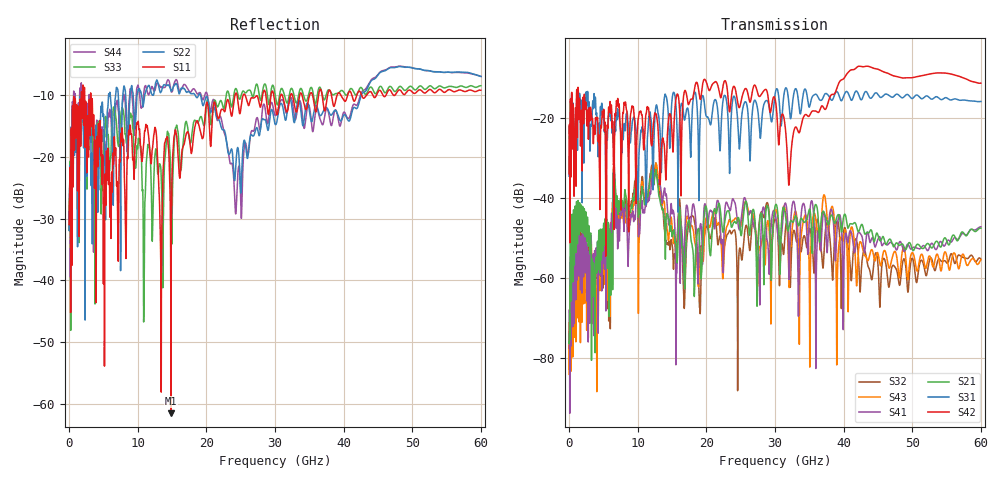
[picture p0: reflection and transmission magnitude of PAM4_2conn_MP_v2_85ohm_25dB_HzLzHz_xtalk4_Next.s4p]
! Info: Touchstone file created by Circ.  Input file=FAB50GbE_2conn_Midplane_Examax_Topo2_v2_85ohm_25dB_HzLzHz.circ
# Hz S RI R 50
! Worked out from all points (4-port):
!   6000 points, 10 MHz to 60 GHz, reference 50 ohm
!   strongest paths, dB at 10 MHz, 15.01 GHz, 30.01 GHz, 45.01 GHz, 60 GHz:
!     S42: -34.0, -24.0, -15.3, -7.9, -11.4
!     S31: -34.6, -15.5, -14.2, -14.2, -16.0
!     S21: -76.0, -49.8, -42.2, -49.4, -47.6
!     S41: -68.1, -44.1, -43.8, -50.4, -47.3
!     S43: -71.3, -47.6, -43.1, -53.9, -55.5
!     S32: -75.1, -51.6, -45.4, -56.8, -55.4
!   lowest |S11| = -61.4 dB at 14.84 GHz (marker M1), VSWR 1.00, Z = 50 + j0.0696 ohm
!   |S11| at or under -10 dB: start of sweep to 1.779 GHz; 3.174 GHz to 24.2 GHz (21.02 GHz wide, 154 % of centre); 25.61 GHz to 28.22 GHz (2.612 GHz wide, 9.71 % of centre)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
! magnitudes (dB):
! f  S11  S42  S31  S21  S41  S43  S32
! 10 MHz  -31.0  -34.0  -34.6  -76.0  -68.1  -71.3  -75.1
! 880 MHz  -10.7  -20.9  -22.9  -42.1  -48.7  -54.5  -48.8
! 3.56 GHz  -13.4  -26.0  -17.4  -56.3  -54.3  -66.3  -65.2
! 6.66 GHz  -18.6  -21.0  -23.3  -35.6  -35.8  -36.7  -36.2
! 14.84 GHz  -61.4  -19.7  -20.5  -47.0  -41.7  -45.1  -50.6
! 24.27 GHz  -9.8  -13.2  -15.9  -46.3  -42.0  -45.1  -49.4
! 60 GHz  -9.3  -11.4  -16.0  -47.6  -47.3  -55.5  -55.4
